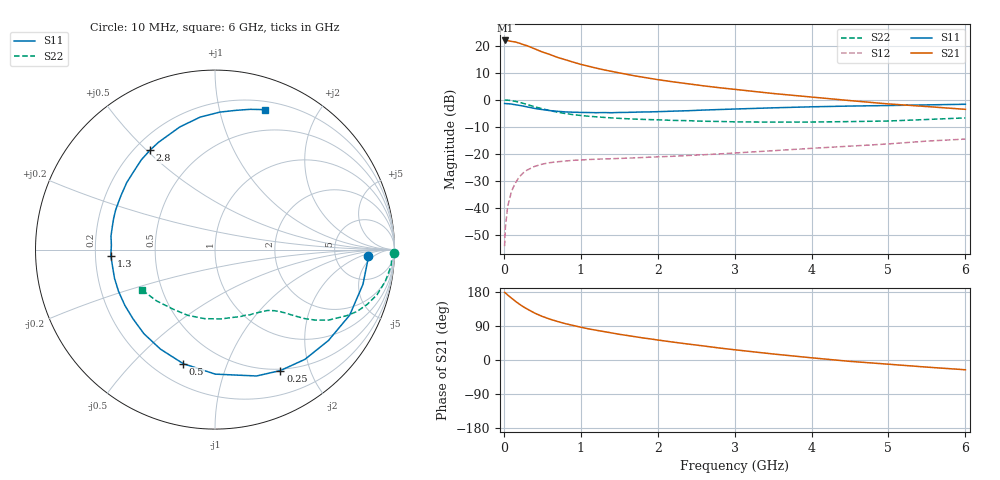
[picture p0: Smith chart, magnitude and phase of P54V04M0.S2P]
! SIEMENS Small Signal Semiconductors
! BFP183
! Si NPN RF Bipolar Junction Transistor in SOT143
! VCE = 4 V  IC = 4 mA
! Common Emitter S-Parameters:  March  1996
# GHz  S  MA  R  50
!  f  S11  S21  S12  S22
! GHz  MAG  ANG  MAG  ANG  MAG  ANG  MAG  ANG
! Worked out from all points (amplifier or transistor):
!   36 points, 10 MHz to 6 GHz, reference 50 ohm
!   highest |S21| = 21.9 dB at 20 MHz (marker M1)
!   |S21| within 3 dB of that: start of sweep to 393.8 MHz
!   unconditionally stable (mu >= 1): 1.712 GHz to 5.62 GHz
!   at 250 MHz: K = 0.18, MSG = 23.7 dB, |S12| = -27.0 dB
!   at 1.4 GHz: K = 0.87, MSG = 16.1 dB, |S12| = -21.7 dB
!   at 6 GHz: K = 0.94, MSG = 5.5 dB, |S12| = -14.5 dB
!   S11 on the Smith chart (normalised r, x): 10 MHz: 12, -3; 250 MHz: 0.48, -1.57; 500 MHz: 0.32, -0.71; 1.3 GHz: 0.26, -0.03; 2.8 GHz: 0.26, +0.51; 6 GHz: 0.28, +1.38
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0.01  0.8557 -2.5  12.34 178.4  0.002 84.5  0.9956 -1.0
0.02  0.8508 -5.5  12.43 177.0  0.0044 87.6  0.9873 -2.1
0.05  0.8468 -13.2  12.33 171.5  0.0108 86.0  0.985 -5.4
0.1  0.8345 -26.0  11.92 163.2  0.0206 74.7  0.9651 -10.6
0.15  0.8099 -38.7  11.64 155.1  0.0294 69.2  0.9369 -15.6
0.2  0.7905 -50.7  11.1 147.7  0.0377 63.7  0.9012 -19.8
0.25  0.7661 -61.6  10.47 140.8  0.0446 59.0  0.8624 -23.6
0.3  0.7412 -71.8  9.957 134.9  0.0504 54.3  0.82 -26.7
0.4  0.6938 -89.9  8.724 123.8  0.0591 46.6  0.745 -31.8
0.5  0.6596 -105.6  7.621 115.0  0.0652 40.9  0.683 -35.1
0.6  0.6324 -118.7  6.826 107.7  0.0694 36.8  0.6321 -37.5
0.7  0.6136 -130.2  6.043 101.5  0.072 33.7  0.5898 -39.2
0.8  0.5977 -139.9  5.479 95.9  0.0743 31.2  0.5582 -40.6
1.1  0.5822 -164.1  4.163 82.2  0.0792 27.3  0.4977 -43.8
1.3  0.5814 -176.6  3.567 75.0  0.0813 25.8  0.4739 -45.9
1.7  0.5909 162.8  2.768 61.7  0.0849 25.7  0.4407 -50.9
2.2  0.6175 142.8  2.144 47.2  0.091 26.6  0.4171 -58.3
2.8  0.6616 123.2  1.672 31.7  0.1005 27.5  0.3989 -69.6
3.5  0.711 106.0  1.307 15.9  0.1153 28.5  0.3877 -85.2
4.5  0.7665 88.0  0.967 -3.6  0.1398 26.3  0.3965 -112.6
5.5  0.8058 75.9  0.751 -18.8  0.1733 22.5  0.4335 -138.8
6  0.8274 70.5  0.667 -25.8  0.1887 18.8  0.4642 -151.0
